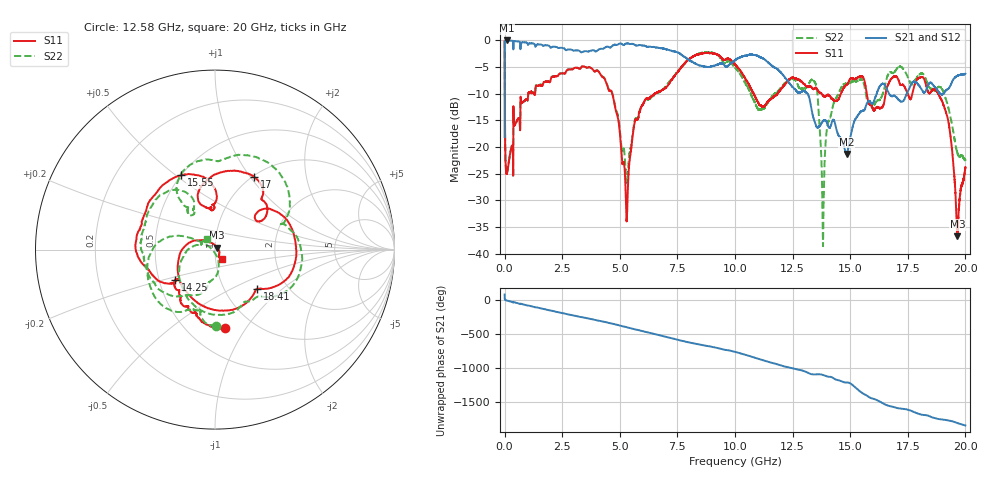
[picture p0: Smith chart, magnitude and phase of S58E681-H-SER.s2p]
!{S58E681}
!Johanson Technology Inc.
!www.johansontechnology.com
!Test Board Conditions:
!Substrate Type  RO4350B
!Substrate Thickness  60 mil
!Substrate Dk  3.66
!TL Type: GCPW
!TL Trace Width  115 mil
!TL Gap  52 mil
!Electrode orientation  Horizontal
!DUT TOPOLOGY	SERIES
!Mounting Pad LxW  55x428 mil
! Created Wed Apr 14 12:00:42 2021
# mhz S ma R 50
! 2 Port Network Data from SP1.SP block
! freq  magS11  angS11  magS21  angS21  magS12  angS12  magS22  angS22
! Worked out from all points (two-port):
!   20001 points, 300 kHz to 20 GHz, reference 50 ohm
!   highest |S21| = -0.01 dB at 99.3 MHz (marker M1); lowest = -21.3 dB at 14.84 GHz (marker M2)
!   |S21| within 3 dB of the highest: 2.433 MHz to 7.78 GHz (7.777 GHz wide, 200 % of centre); 10.31 GHz to 11.03 GHz (723.3 MHz wide, 6.78 % of centre)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
!   lowest |S11| = -36.7 dB at 19.65 GHz (marker M3), VSWR 1.03, Z = 51 + j1.1 ohm
!   |S11| at or under -10 dB: 4.67 GHz to 6.505 GHz (1.835 GHz wide, 32.8 % of centre); 10.81 GHz to 11.84 GHz (1.033 GHz wide, 9.12 % of centre); 18.82 GHz to end of sweep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
!   |S22| runs from -38.6 to -0.1 dB; largest |S21 - S12| = 0.011
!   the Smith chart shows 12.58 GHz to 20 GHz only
!   S11 on the Smith chart (normalised r, x): 12.58 GHz: 0.75, -0.81; 14.25 GHz: 0.60, -0.22; 15.55 GHz: 0.50, +0.52; 17 GHz: 1.02, +1.05; 18.41 GHz: 1.42, -0.69; 20 GHz: 1.08, -0.11
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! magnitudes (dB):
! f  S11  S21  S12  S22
! 300 kHz  -0.1  -18.1  -18.1  -0.1
! 99.3 MHz  -24.9  0.0  0.0  -24.9
! 786.3 MHz  -11.6  -0.3  -0.4  -11.7
! 3.334 GHz  -5.0  -2.3  -2.3  -5.0
! 4.667 GHz  -10.0  -1.0  -1.0  -9.8
! 5.298 GHz  -33.8  -0.6  -0.6  -26.7
! 5.671 GHz  -15.0  -0.9  -0.9  -14.8
! 6.667 GHz  -9.6  -1.4  -1.4  -9.8
! 10 GHz  -4.5  -3.7  -3.7  -5.1
! 11.07 GHz  -12.1  -3.1  -3.1  -13.0
! 12.58 GHz  -7.1  -9.1  -9.0  -7.4
! 13.33 GHz  -8.9  -13.2  -13.1  -7.4
! 13.82 GHz  -10.3  -15.1  -15.1  -38.1
! 14.25 GHz  -11.0  -14.9  -14.7  -12.2
! 14.84 GHz  -8.3  -21.3  -21.3  -8.1
! 15.55 GHz  -6.8  -13.2  -13.2  -7.6
! 16.67 GHz  -8.1  -9.8  -9.9  -6.2
! 17 GHz  -6.8  -10.7  -10.7  -5.5
! 18.41 GHz  -9.9  -8.2  -8.2  -8.6
! 19.21 GHz  -14.2  -9.2  -9.1  -11.8
! 19.65 GHz  -36.7  -6.7  -6.6  -21.0
! 20 GHz  -23.8  -6.3  -6.2  -22.5
